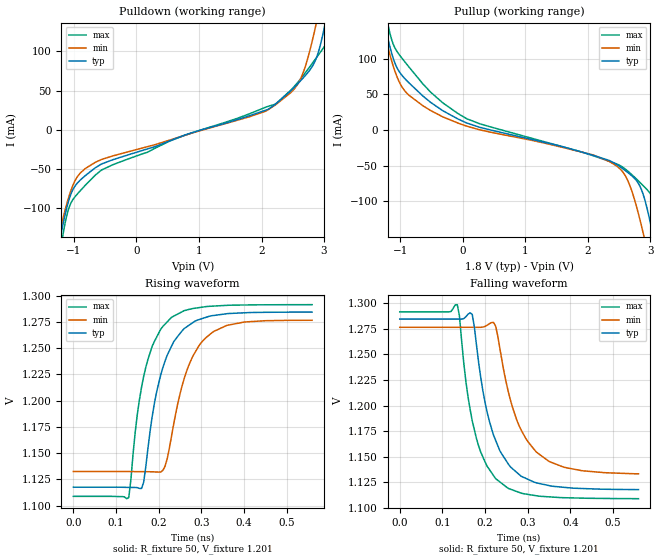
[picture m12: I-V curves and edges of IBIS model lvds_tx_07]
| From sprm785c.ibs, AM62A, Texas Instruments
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|   MODEL lvds_tx_07
[Model] lvds_tx_07
Model_type Output
C_comp 1.573p 1.644p 1.493p
Vmeas = 1.2
Vref = 1.2V
Rref = 50
Cref = 0.5pF
[Model Spec]
[Temperature Range]  40 150 -40
[Voltage Range] 1.8 1.62 1.98
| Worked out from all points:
|   slope of the pulldown table from 0 to 0.27 V, typ, clamps not added: 41.8 ohm
|   slope of the pullup table from 0 to 0.27 V, typ, clamps not added: 31.7 ohm
|   rising waveform, R_fixture 50, V_fixture 1.201: 20-80 % time 55.4ps typ, 59.8ps min, 49.2ps max; typ from 1.12 V to 1.28 V
|   falling waveform, R_fixture 50, V_fixture 1.201: 20-80 % time 59.3ps typ, 67.9ps min, 52.4ps max; typ from 1.28 V to 1.12 V
[Pulldown]
-1.71V    -379mA     -326.5mA   -450.1mA
-1.245V   -150.1mA   -137.8mA   -169.1mA
-1.166V   -117.5mA   -110.5mA   -129.8mA
-1.013V   -75.87mA   -70.25mA   -88.69mA
-817.9mV  -58.4mA    -49.39mA   -70.74mA
-374.4mV  -38.05mA   -33.19mA   -44.41mA
2.064V    25.04mA    23.71mA    28.77mA
2.576V    58.58mA    57.94mA    60.27mA
2.861V    88.61mA    130.7mA    90.3mA
3.015V    134.5mA    189.1mA    107.5mA
3.136V    187.3mA    238.6mA    132mA
3.511V    373.4mA    396.1mA    334.9mA
[Pullup]
-1.711V   373.4mA    320.3mA    445.5mA
-1.273V   158.7mA    142mA      183.9mA
-1.193V   126.4mA    114.1mA    146mA
-1.014V   81.17mA    66.68mA    105.1mA
-639.2mV  47.48mA    33.83mA    64.45mA
62.91mV   9.544mA    5.151mA    15.55mA
2.343V    -42.99mA   -44.42mA   -44.08mA
2.634V    -59.52mA   -70.36mA   -57.51mA
2.882V    -90.02mA   -143.8mA   -78.08mA
3.03V     -143.2mA   -201.3mA   -93.79mA
3.172V    -208.9mA   -260mA     -141.8mA
3.51V     -379mA     -402.7mA   -338mA
[Ramp]
dV/dt_r .1/55.543p .087/59.842p .11/49.266p
dV/dt_f .1/59.654p .087/68.933p .11/52.557p
[Rising Waveform]
R_fixture = 50
V_fixture = 1.201
V_fixture_min = 1.205
V_fixture_max = 1.2
0s        1.117V     1.132V     1.109V
130ps     1.117V     1.132V     1.108V
150ps     1.117V     1.132V     1.187V
170ps     1.137V     1.132V     1.232V
195ps     1.208V     1.132V     1.26V
215ps     1.238V     1.137V     1.273V
230ps     1.252V     1.165V     1.279V
270ps     1.271V     1.233V     1.287V
325ps     1.281V     1.265V     1.29V
560ps     1.284V     1.277V     1.291V
[Falling Waveform]
R_fixture = 50
V_fixture = 1.201
V_fixture_min = 1.205
V_fixture_max = 1.2
0s        1.285V     1.277V     1.292V
135ps     1.285V     1.277V     1.299V
155ps     1.287V     1.277V     1.224V
170ps     1.289V     1.277V     1.185V
195ps     1.214V     1.277V     1.15V
225ps     1.166V     1.278V     1.128V
265ps     1.138V     1.198V     1.117V
320ps     1.124V     1.155V     1.112V
390ps     1.12V      1.139V     1.11V
560ps     1.118V     1.133V     1.109V
